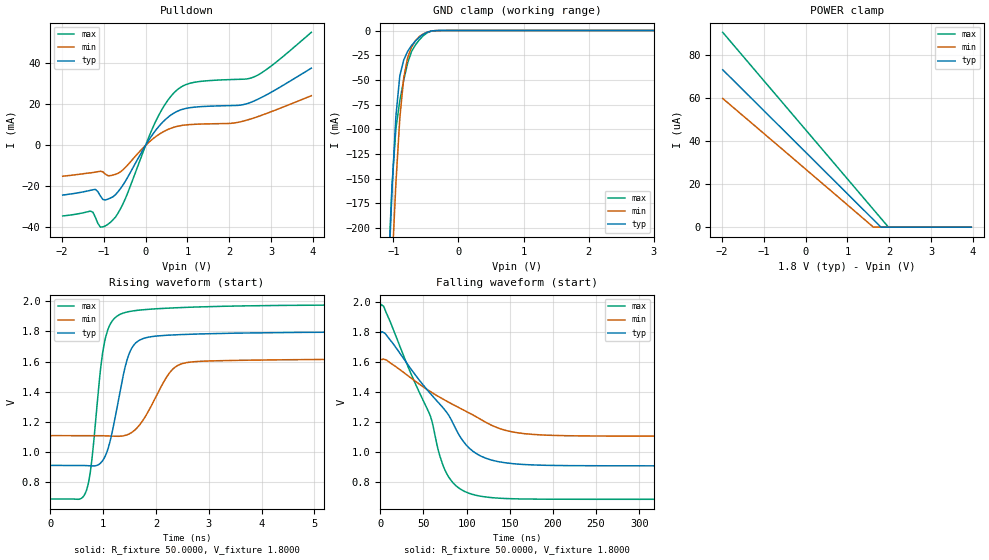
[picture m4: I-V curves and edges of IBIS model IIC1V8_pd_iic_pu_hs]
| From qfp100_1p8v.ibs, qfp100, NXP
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[Model] IIC1V8_pd_iic_pu_hs
|   Model IIC1V8_pd_iic_pu_hs
| This model was characterised for following simulation conditions:
| External (pad) voltage:
|   - Typ: 1.8V,   - Min: 1.62V,   - Max: 1.98V
| Library cells for typ/min/max conditions are connected as defined below:
|  IO - External Pad
|  A - Core Input
|  EN - Output Buffer Enable
|  BOOST - vdde
|  ECS - vdd
|  EGP - gnd
|  ENZI - vdd
|  EPD - vdd
|  EPUN - vdd
|  SSEL - vdd
|  ZI - NC
|  ZIF - NC
|  gnd - gnd
|  gnde - gnde
|  vdd - vdd
|  vdde - vdde
| All other pins connected to ground
Model_type I/O_open_drain
Polarity   Non-Inverting
Enable   Active-Low
Vinl =   0.5400V
Vinh =   1.2600V
Vmeas =  0.9000V
Cref =   0.0F
Rref =   1000.000
Vref =   1.8000V
C_comp   3.6136pF   3.4665pF   3.7543pF
|C_comp_pullup   0.9376pF   0.9156pF   0.9440pF
|C_comp_pulldown   2.3254pF   2.4783pF   2.1797pF
[Model Spec]
| variable   typ   min   max
Vinh   0.5400V   0.4860V   0.5940V
Vinl   1.2600V   1.1340V   1.3860V
Vmeas   0.9000V   0.8100V   0.9900V
Vref   1.8000V   1.6200V   1.9800V
Cref   0.0F   0.0F   0.0F
Rref   1.0000k   1.0000k   1.0000k
[Temperature Range]   25.0000   0.1250k   -40.0000
[Voltage Range]   1.8000V   1.6200V   1.9800V
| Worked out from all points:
|   slope of the pulldown table from 0 to 0.27 V, typ, clamps not added: 33.4 ohm
|   GND clamp passes 1 mA (typ) near -0.44 V on its own axis
|   rising waveform, R_fixture 50.0000, V_fixture 1.8000: 20-80 % time 318ps typ, 487ps min, 235ps max; typ from 0.91 V to 1.8 V
|   falling waveform, R_fixture 50.0000, V_fixture 1.8000: 20-80 % time 66.9ns typ, 88.6ns min, 48.9ns max; typ from 1.8 V to 0.91 V
[Pulldown]
|Voltage   I(typ)   I(min)   I(max)
-1.98V    -24.22mA   -15.04mA   -34.42mA
-1.32V    -21.94mA   -13.4mA    -32.06mA
-1.2V     -21.45mA   -13.05mA   -35.06mA
-1.08V    -24.63mA   -12.6mA    -39.9mA
-900mV    -26.23mA   -14.78mA   -38.53mA
-720mV    -24.07mA   -14.13mA   -34.99mA
-540mV    -19.33mA   -11.9mA    -28.53mA
300mV     8.856mA    5.096mA    14.12mA
720mV     16.26mA    9.117mA    26.48mA
1.14V     18.6mA     10.26mA    30.69mA
2.58V     21.55mA    13.34mA    33.32mA
3.96V     37.7mA     24.26mA    55.17mA
[GND_clamp]
|Voltage   I(typ)   I(min)   I(max)
-1.98V    -2.104A    -2.075A    -2.136A
-1.08V    -259.3mA   -333mA     -246.9mA
-1.02V    -161.8mA   -238.7mA   -157.1mA
-960mV    -86.75mA   -154.7mA   -99.47mA
-900mV    -45.96mA   -88.82mA   -71.06mA
-840mV    -29.91mA   -48mA      -50.26mA
-780mV    -21.16mA   -27.65mA   -32.99mA
-720mV    -15.17mA   -16.88mA   -21.27mA
-660mV    -10.57mA   -10.24mA   -14.57mA
-540mV    -3.796mA   -3.405mA   -5.301mA
-300mV    -21.69uA   -40.85uA   -23.15uA
3.96V     0A         0A         0A
[POWER_clamp]
|Voltage   I(typ)   I(min)   I(max)
-1.98V    73.06uA    59.72uA    90.42uA
1.62V     3.484uA    0A         8.225uA
1.8V      0A         0A         4.113uA
1.98V     0A         0A         0A
3.96V     0A         0A         0A
[Ramp]
| variable   typ   min   max
dV/dt_r  0.5332/0.3184n   0.3066/0.4867n   0.7749/0.2353n
dV/dt_f  0.5332/66.8941n   0.3065/88.5976n   0.7749/48.9326n
R_load = 50.0000
[Rising Waveform]
R_fixture= 50.0000
V_fixture= 1.8000
V_fixture_min= 1.6200
V_fixture_max= 1.9800
|time   V(typ)   V(min)   V(max)
0s        910.3mV    1.108V     687.5mV
675ps     909mV      1.108V     735mV
774.6ps   906.6mV    1.108V     908.9mV
1.009ns   951.5mV    1.107V     1.696V
1.274ns   1.313V     1.104V     1.904V
1.48ns    1.64V      1.117V     1.931V
1.77ns    1.754V     1.218V     1.944V
2.479ns   1.779V     1.584V     1.959V
5.427ns   1.795V     1.615V     1.975V
1us       1.799V     1.619V     1.979V
[Falling Waveform]
R_fixture= 50.0000
V_fixture= 1.8000
V_fixture_min= 1.6200
V_fixture_max= 1.9800
|time   V(typ)   V(min)   V(max)
0s        1.799V     1.619V     1.979V
4.129ns   1.799V     1.622V     1.972V
58.3ns    1.391V     1.405V     1.238V
68.89ns   1.323V     1.368V     978.3mV
76.97ns   1.267V     1.342V     858.8mV
95.13ns   1.082V     1.287V     748mV
110.6ns   994.8mV    1.24V      714.6mV
145.4ns   930.7mV    1.147V     692.8mV
203.1ns   913.1mV    1.113V     688.1mV
1us       910.4mV    1.108V     687.5mV
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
